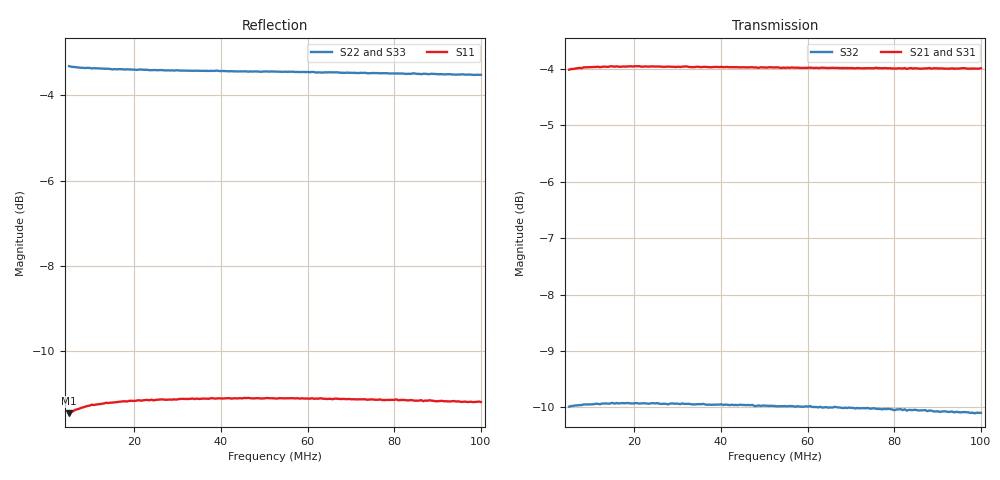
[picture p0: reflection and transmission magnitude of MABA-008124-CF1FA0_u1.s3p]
#	MHz	S	dB	R	75
!FREQ	R1	I1	R2	I2	R3	I3
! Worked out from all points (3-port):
!   201 points, 5 MHz to 100 MHz, reference 75 ohm
!   strongest paths, dB at 5 MHz, 28.75 MHz, 52.5 MHz, 76.25 MHz, 100 MHz:
!     S21: -4.0, -4.0, -4.0, -4.0, -4.0
!     S31: -4.0, -4.0, -4.0, -4.0, -4.0
!     S32: -10.0, -9.9, -10.0, -10.0, -10.1
!   lowest |S11| = -11.5 dB at 5 MHz (marker M1), VSWR 1.73, Z = 128 + j13.3 ohm
!   |S11| at or under -10 dB: start of sweep to end of sweep
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5  -11.46 10.4  -4.02 -178.3  -4.02 1.8
   -4.02 -178.3  -3.32 178.3  -9.99 -178.2
   -4.02 1.8  -9.99 -178.2  -3.32 178.5
6.9  -11.36 7.7  -4.00 -178.9  -3.99 1.1
     -3.99 -179.0  -3.35 178.3  -9.96 -178.8
     -3.99 1.1  -9.96 -178.9  -3.33 178.4
9.75  -11.27 5.3  -3.97 -179.7  -3.97 0.4
      -3.97 -179.8  -3.36 178.2  -9.93 -179.6
      -3.97 0.4  -9.94 -179.6  -3.35 178.4
13.075  -11.22 3.6  -3.97 179.6  -3.96 -0.3
        -3.96 179.6  -3.38 178.1  -9.92 179.7
        -3.96 -0.3  -9.93 179.8  -3.37 178.3
13.55  -11.21 3.5  -3.96 179.6  -3.95 -0.2
       -3.97 179.5  -3.38 178.0  -9.93 179.8
       -3.95 -0.2  -9.93 179.7  -3.37 178.3
17.35  -11.18 2.1  -3.96 179.0  -3.95 -0.8
       -3.96 178.9  -3.39 177.8  -9.91 179.2
       -3.95 -0.8  -9.92 179.2  -3.38 178.1
31.6  -11.12 -0.9  -3.96 177.4  -3.96 -2.4
      -3.96 177.1  -3.42 176.7  -9.93 177.6
      -3.96 -2.4  -9.94 177.6  -3.40 177.1
52.5  -11.11 -3.9  -3.98 175.3  -3.98 -4.4
      -3.98 174.9  -3.45 175.0  -9.96 175.6
      -3.98 -4.4  -9.97 175.6  -3.40 175.5
75.775  -11.14 -6.8  -3.97 173.1  -4.01 -6.6
        -3.98 172.4  -3.48 173.1  -10.02 173.6
        -4.01 -6.6  -10.02 173.5  -3.42 173.7
100  -11.19 -9.4  -3.97 170.8  -4.04 -8.7
     -3.99 170.1  -3.52 171.1  -10.09 171.5
     -4.04 -8.7  -10.09 171.6  -3.42 171.9
